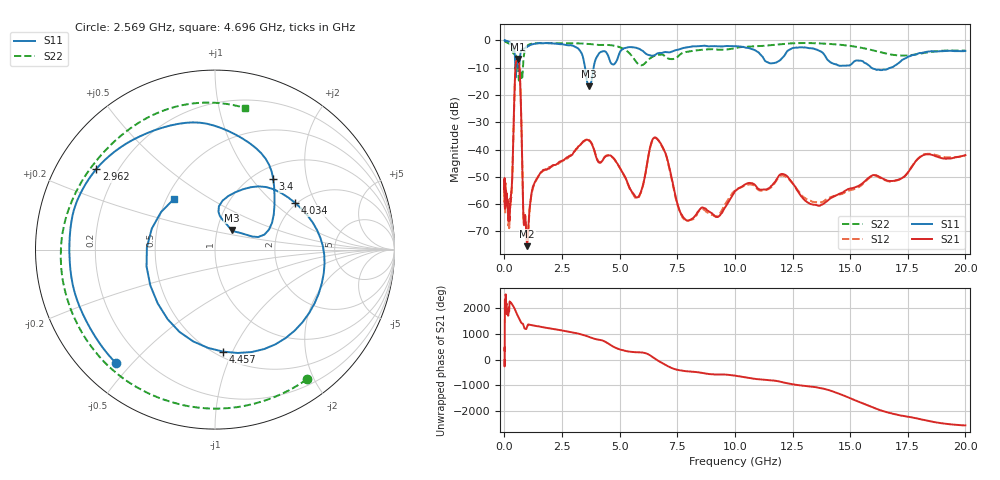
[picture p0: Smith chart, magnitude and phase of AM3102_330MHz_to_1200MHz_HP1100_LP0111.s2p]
! Date/Time: Tue, Sep 11, 2018 5:21 PM
! Network Analyzer: Agilent Technologies E8362B Rev: A.07.50.63
! Sweep from 0.010 to 20.000 GHz, 1601 Points, Sweep Type: LOG
! Power Supply: 4.949 V, 0.001 A
# Hz S DB R 50
!freq MagS11 AngS11 MagS21 AngS21 MagS12 AngS12 MagS22 AngS22
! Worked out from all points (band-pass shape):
!   1601 points, 10 MHz to 20 GHz, reference 50 ohm
!   highest |S21| = -6.82 dB at 591.9 MHz (marker M1); lowest = -75.4 dB at 988.7 MHz (marker M2)
!   |S21| within 3 dB of the highest: 482.5 MHz to 652.6 MHz (170.1 MHz wide, 30 % of centre)
!   lowest |S11| = -16.9 dB at 3.668 GHz (marker M3), VSWR 1.33, Z = 58.6 + j13.1 ohm
!   |S11| at or under -10 dB: 472.4 MHz to 522 MHz (49.6 MHz wide, 9.98 % of centre); 3.501 GHz to 3.87 GHz (369.5 MHz wide, 10 % of centre); 15.92 GHz to 16.77 GHz (852.4 MHz wide, 5.22 % of centre)
!   |S22| runs from -14.8 to -0.2 dB; largest |S21 - S12| = 0.0073
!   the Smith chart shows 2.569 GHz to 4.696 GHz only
!   S11 on the Smith chart (normalised r, x): 2.569 GHz: 0.11, -0.45; 2.962 GHz: 0.12, +0.30; 3.4 GHz: 1.21, +1.29; 4.034 GHz: 1.96, +1.39; 4.457 GHz: 0.55, -0.92; 4.696 GHz: 0.55, +0.36
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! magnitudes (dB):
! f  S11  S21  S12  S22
! 10 MHz  0.0  -51.1  -54.3  -0.2
! 35.55 MHz  -0.1  -59.9  -61.6  -0.4
! 126.4 MHz  -0.3  -58.3  -59.8  -0.9
! 202.3 MHz  -0.6  -63.9  -68.3  -1.2
! 307.3 MHz  -1.4  -55.4  -56.2  -2.3
! 447.2 MHz  -4.5  -16.9  -16.9  -4.6
! 591.9 MHz  -8.5  -6.8  -6.9  -10.1
! 695.6 MHz  -4.9  -17.6  -17.7  -10.4
! 833.3 MHz  -3.1  -66.0  -66.0  -6.6
! 988.7 MHz  -2.4  -75.4  -73.2  -2.0
! 1.59 GHz  -1.0  -48.3  -48.4  -1.0
! 2.569 GHz  -1.5  -44.0  -43.9  -1.1
! 2.962 GHz  -1.9  -41.7  -41.3  -1.1
! 3.4 GHz  -5.8  -37.2  -37.3  -1.2
! 3.668 GHz  -16.9  -36.7  -36.4  -1.3
! 4.034 GHz  -5.7  -43.9  -43.7  -1.7
! 4.457 GHz  -4.9  -42.2  -42.1  -1.7
! 4.696 GHz  -8.8  -42.8  -42.9  -1.9
! 5.652 GHz  -2.6  -56.8  -57.3  -7.1
! 6.58 GHz  -5.1  -35.7  -35.9  -5.5
! 7.995 GHz  -2.4  -66.0  -66.0  -4.1
! 20 GHz  -3.9  -42.0  -42.4  -3.7
